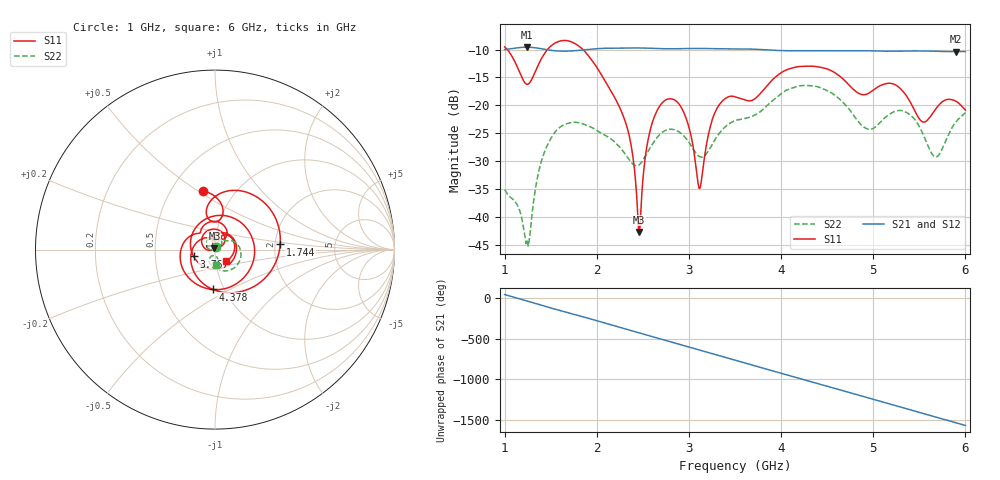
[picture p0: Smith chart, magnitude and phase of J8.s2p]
!Agilent Technologies,E8364B,MY43040528,A.07.50.67
!Agilent E8364B: A.07.50.67
!Date: Sunday, March 01, 2026 18:31:35
!Correction: S11(Full 2 Port(1,2))
!S21(Full 2 Port(1,2))
!S12(Full 2 Port(1,2))
!S22(Full 2 Port(1,2))
!S2P File: Measurements: S11, S21, S12, S22:
# Hz S  dB  R 50
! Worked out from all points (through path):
!   451 points, 1 GHz to 6 GHz, reference 50 ohm
!   highest |S21| = -9.59 dB at 1.244 GHz (marker M1); lowest = -10.4 dB at 5.9 GHz (marker M2)
!   group delay of S21, straight-line fit = 897 ps
!   lowest |S11| = -42.7 dB at 2.456 GHz (marker M3), VSWR 1.01, Z = 49.7 + j0.654 ohm
!   |S11| at or under -10 dB: 1.028 GHz to 1.466 GHz (437.4 MHz wide, 35.1 % of centre); 1.849 GHz to end of sweep
!   |S22| runs from -45.2 to -16.4 dB; largest |S21 - S12| = 0.0014
!   S11 on the Smith chart (normalised r, x): 1 GHz: 0.71, +0.52; 1.744 GHz: 2.13, +0.14; 3.767 GHz: 0.78, -0.06; 4.378 GHz: 0.88, -0.41; 6 GHz: 1.12, -0.15
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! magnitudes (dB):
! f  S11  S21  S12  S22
! 1 GHz  -9.5  -10.0  -10.0  -35.1
! 1.244 GHz  -16.2  -9.6  -9.6  -44.0
! 1.433 GHz  -10.7  -10.0  -10.0  -28.3
! 1.744 GHz  -8.8  -10.2  -10.3  -23.0
! 1.844 GHz  -9.9  -10.1  -10.1  -23.3
! 2.311 GHz  -23.0  -9.7  -9.8  -28.8
! 2.456 GHz  -42.7  -9.7  -9.8  -30.7
! 2.556 GHz  -26.2  -9.8  -9.8  -28.2
! 2.667 GHz  -20.5  -9.8  -9.8  -25.5
! 2.922 GHz  -20.5  -9.8  -9.9  -25.1
! 3.111 GHz  -34.9  -9.8  -9.8  -29.1
! 3.278 GHz  -21.4  -9.9  -9.9  -26.3
! 3.5 GHz  -18.5  -9.9  -9.9  -22.7
! 3.767 GHz  -18.0  -10.0  -10.0  -21.2
! 4.344 GHz  -13.0  -10.2  -10.2  -16.5
! 4.378 GHz  -13.0  -10.2  -10.2  -16.6
! 4.933 GHz  -18.0  -10.2  -10.2  -24.2
! 5.167 GHz  -16.0  -10.3  -10.3  -21.7
! 5.533 GHz  -22.9  -10.3  -10.3  -24.9
! 5.678 GHz  -20.6  -10.3  -10.3  -29.2
! 5.9 GHz  -19.3  -10.4  -10.4  -22.9
! 6 GHz  -20.8  -10.4  -10.4  -21.3
